VAR_GLOBAL CONSTANT
		N_AXES			: USINT := 2;
	END_VAR
	VAR_GLOBAL
		gCommunicationReady	: BOOL := FALSE; (* Global indicator for Tria-Link and axes readiness *)
		gReset				: BOOL := FALSE; (* Global handle to reset axes errors *)
		gEnable				: BOOL := FALSE; (* Global handle to enable/disable axes *)
	
		gTrialink			: Triamec.TL_Trialink2; (* The Trialink adapter *)
		gAxes				: ARRAY [1..N_AXES] OF Triamec.TL_Axis2; (* The Triamec Axis objects *)
		{attribute 'contextName' := 'TASK_FAST'}
		gNciAxes			: ARRAY [1..N_AXES] OF TL_NCI_Axis; (* Link to the NC pathplanner *)
		
		motorTemperature1	: Triamec.TL_MC_RegisterRead;
		publish1			: Triamec.TL_publishSlave2Master;
	END_VAR
